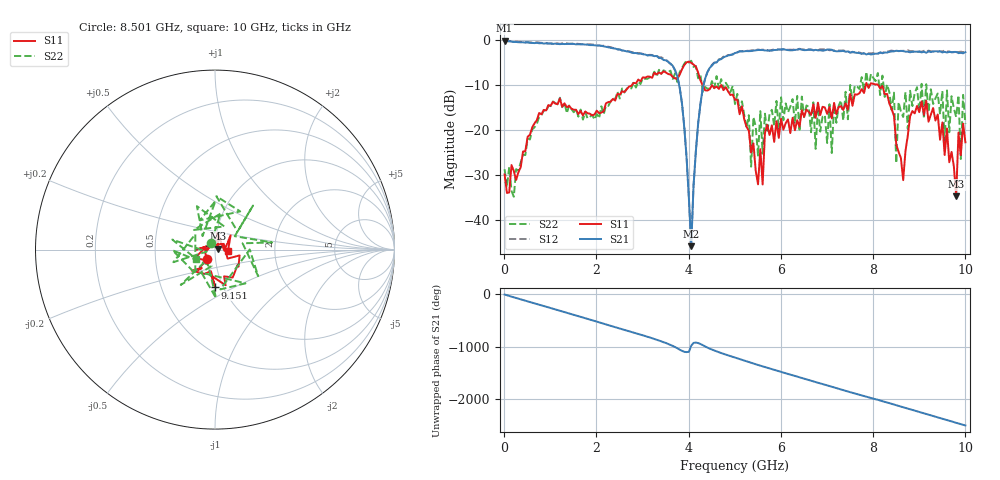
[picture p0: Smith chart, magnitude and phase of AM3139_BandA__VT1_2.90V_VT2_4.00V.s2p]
! Date/Time: Tue, Nov 13, 2018 4:57 PM
! Network Analyzer: Agilent Technologies E8364B Rev: A.07.50.67
! Sweep from 0.010 to 10.000 GHz, 201 Points, Sweep Type: LIN
! Power Supply: 2.901 V, 0.000 A
# Hz S DB R 50
!freq MagS11 AngS11 MagS21 AngS21 MagS12 AngS12 MagS22 AngS22
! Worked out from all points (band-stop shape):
!   201 points, 10 MHz to 10 GHz, reference 50 ohm
!   highest |S21| = -0.24 dB at 10 MHz (marker M1); lowest = -45.8 dB at 4.056 GHz (marker M2)
!   |S21| within 3 dB of the highest: start of sweep to 3.022 GHz; 4.964 GHz to 7.846 GHz (2.883 GHz wide, 45 % of centre)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
!   lowest |S11| = -34.7 dB at 9.8 GHz (marker M3), VSWR 1.04, Z = 51.8 + j0.633 ohm
!   |S11| at or under -10 dB: start of sweep to 2.774 GHz; 4.298 GHz to 7.843 GHz (3.544 GHz wide, 58.4 % of centre); 8.106 GHz to end of sweep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
!   |S22| runs from -34.8 to -4.6 dB; largest |S21 - S12| = 0.031
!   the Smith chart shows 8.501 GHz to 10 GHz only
!   S11 on the Smith chart (normalised r, x): 8.501 GHz: 0.91, -0.10; 9.151 GHz: 0.92, -0.40; 10 GHz: 1.16, -0.02
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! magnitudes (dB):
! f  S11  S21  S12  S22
! 10 MHz  -29.9  -0.2  -0.2  -28.7
! 1.708 GHz  -16.8  -1.0  -1.0  -17.7
! 3.357 GHz  -7.3  -4.1  -3.9  -6.7
! 3.806 GHz  -7.7  -10.7  -10.6  -7.2
! 4.056 GHz  -5.1  -45.8  -45.6  -4.7
! 4.306 GHz  -10.2  -10.8  -10.7  -11.6
! 5.005 GHz  -13.3  -2.9  -2.8  -14.3
! 5.505 GHz  -32.1  -2.3  -2.2  -25.7
! 5.704 GHz  -18.9  -2.4  -2.3  -20.6
! 6.703 GHz  -14.3  -2.4  -2.3  -13.9
! 7.103 GHz  -17.5  -2.2  -2.3  -25.1
! 7.502 GHz  -12.0  -2.9  -2.8  -10.0
! 8.352 GHz  -14.2  -2.7  -2.5  -11.7
! 8.452 GHz  -16.9  -2.6  -2.5  -11.8
! 8.501 GHz  -23.2  -2.4  -2.4  -27.4
! 8.551 GHz  -24.9  -2.5  -2.5  -13.9
! 9.151 GHz  -13.5  -2.9  -2.7  -9.9
! 9.8 GHz  -34.7  -2.7  -2.7  -17.1
! 9.85 GHz  -20.6  -3.0  -2.7  -12.3
! 9.9 GHz  -25.7  -2.9  -2.6  -26.5
! 9.95 GHz  -18.6  -3.0  -2.8  -12.2
! 10 GHz  -22.8  -2.8  -2.7  -18.6
